{attribute 'GUID' := '56AA2C35-D736-E752-6308-29B40FF3D0B1'}
TYPE DUT_BalluffSmartLightOut :
STRUCT
			 {attribute 'GUID' := '18071995-0000-0000-0000-000000000010}
		MDP5001_6220_Segment_1_color_IECCONF_IECCONF_Background_color_IECCONF_IECCONF_LED3_1_Bit0 : BIT;
		 {attribute 'GUID' := '18071995-0000-0000-0000-000000000010}
		MDP5001_6220_Segment_1_color_IECCONF_IECCONF_Background_color_IECCONF_IECCONF_LED3_1_Bit1 : BIT;
		 {attribute 'GUID' := '18071995-0000-0000-0000-000000000010}
		MDP5001_6220_Segment_1_color_IECCONF_IECCONF_Background_color_IECCONF_IECCONF_LED3_1_Bit2 : BIT;
		MDP5001_6220_Segment_1_blink_IECCONF_IECCONF_dominant_IECCONF_IECCONF_LED4 : BIT;
		 {attribute 'GUID' := '18071995-0000-0000-0000-000000000010}
		MDP5001_6220_Segment_2_color_IECCONF_IECCONF_Running_color_IECCONF_IECCONF_LED7_5_Bit0 : BIT;
		 {attribute 'GUID' := '18071995-0000-0000-0000-000000000010}
		MDP5001_6220_Segment_2_color_IECCONF_IECCONF_Running_color_IECCONF_IECCONF_LED7_5_Bit1 : BIT;
		 {attribute 'GUID' := '18071995-0000-0000-0000-000000000010}
		MDP5001_6220_Segment_2_color_IECCONF_IECCONF_Running_color_IECCONF_IECCONF_LED7_5_Bit2 : BIT;
		MDP5001_6220_Segment_2_blink_IECCONF_IECCONF_dominant_IECCONF_IECCONF_LED8 : BIT;
		 {attribute 'GUID' := '18071995-0000-0000-0000-000000000010}
		MDP5001_6220_Segment_3_color_IECCONF_IECCONF_LED11_9_Bit0 : BIT;
		 {attribute 'GUID' := '18071995-0000-0000-0000-000000000010}
		MDP5001_6220_Segment_3_color_IECCONF_IECCONF_LED11_9_Bit1 : BIT;
		 {attribute 'GUID' := '18071995-0000-0000-0000-000000000010}
		MDP5001_6220_Segment_3_color_IECCONF_IECCONF_LED11_9_Bit2 : BIT;
		MDP5001_6220_Segment_3_blink_IECCONF_IECCONF_dominant_IECCONF_IECCONF_LED12 : BIT;
		 {attribute 'GUID' := '18071995-0000-0000-0000-000000000010}
		MDP5001_6220_Segment_4_color_IECCONF_IECCONF_LED15_13_Bit0 : BIT;
		 {attribute 'GUID' := '18071995-0000-0000-0000-000000000010}
		MDP5001_6220_Segment_4_color_IECCONF_IECCONF_LED15_13_Bit1 : BIT;
		 {attribute 'GUID' := '18071995-0000-0000-0000-000000000010}
		MDP5001_6220_Segment_4_color_IECCONF_IECCONF_LED15_13_Bit2 : BIT;
		MDP5001_6220_Segment_4_blink_IECCONF_IECCONF_dominant_IECCONF_IECCONF_LED16 : BIT;
		 {attribute 'GUID' := '18071995-0000-0000-0000-000000000010}
		MDP5001_6220_Segment_5_color_IECCONF_IECCONF_LED19_17_Bit0 : BIT;
		 {attribute 'GUID' := '18071995-0000-0000-0000-000000000010}
		MDP5001_6220_Segment_5_color_IECCONF_IECCONF_LED19_17_Bit1 : BIT;
		 {attribute 'GUID' := '18071995-0000-0000-0000-000000000010}
		MDP5001_6220_Segment_5_color_IECCONF_IECCONF_LED19_17_Bit2 : BIT;
		MDP5001_6220_Segment_5_blink_IECCONF_IECCONF_dominant_IECCONF_IECCONF_LED20 : BIT;
		 {attribute 'GUID' := '18071995-0000-0000-0000-000000000010}
		MDP5001_6220_Buzzer_type_Bit0 : BIT;
		 {attribute 'GUID' := '18071995-0000-0000-0000-000000000010}
		MDP5001_6220_Buzzer_type_Bit1 : BIT;
		BuzzerState : BIT;
		 {attribute 'GUID' := '18071995-0000-0000-0000-000000000010}
		MDP5001_6220_Operating_mode_Bit0 : BIT;
		 {attribute 'GUID' := '18071995-0000-0000-0000-000000000010}
		MDP5001_6220_Operating_mode_Bit1 : BIT;
		 {attribute 'GUID' := '18071995-0000-0000-0000-000000000010}
		MDP5001_6220_Operating_mode_Bit2 : BIT;
		 {attribute 'GUID' := '18071995-0000-0000-0000-000000000010}
		MDP5001_6220_Operating_mode_Bit3 : BIT;
		MDP5001_6220_Runlight_running_direction : BIT;
		MDP5001_6220_Sync_Start : BIT;
		MDP5001_6220_Sync_Impulse : BIT;
		 {attribute 'hide'}
		_reserved1 : BIT;
		 {attribute 'hide'}
		_reserved2 : BIT;
		MDP5001_6220_Number_of_segments_IECCONF_IECCONF_Level_type : BYTE;
		MDP5001_6220_Blinking_mode_IECCONF_IECCONF_Level_value_low_byte : BYTE;
		MDP5001_6220_Blinking_frequency_IECCONF_IECCONF_Level_value_high_byte_IECCONF_IECCONF_Running_speed : BYTE;
		MDP5001_6220_Buzzer_Volume : BYTE;
END_STRUCT
END_TYPE
